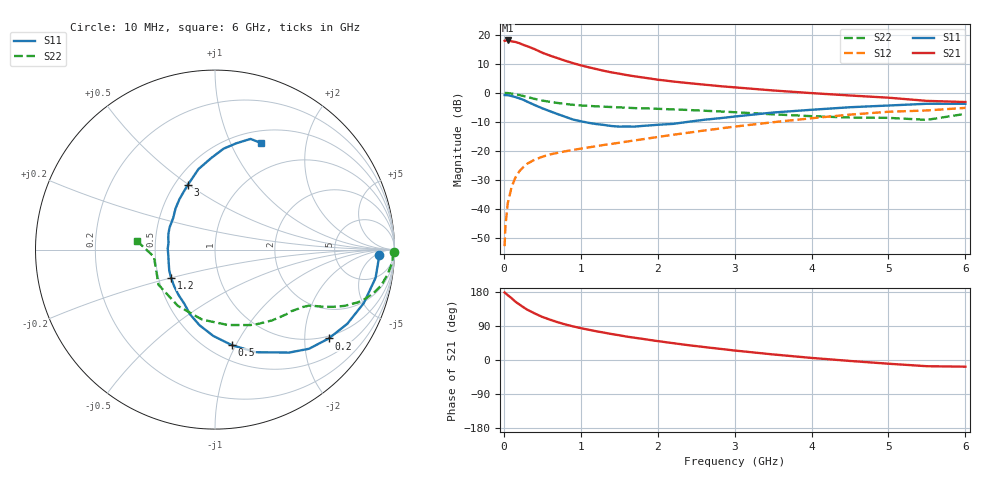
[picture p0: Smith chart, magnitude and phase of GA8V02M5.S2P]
! Infineon Technologies  Discrete & RF Semiconductors
! BF775
! Si NPN RF Bipolar Junction Transistor in SOT23
! VCE = 8 V  IC = 2.5 mA
! Common Emitter S-Parameters:  May  1996
# GHz  S  MA  R  50
!  f  S11  S21  S12  S22
! GHz  MAG  ANG  MAG  ANG  MAG  ANG  MAG  ANG
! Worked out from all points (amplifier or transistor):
!   36 points, 10 MHz to 6 GHz, reference 50 ohm
!   highest |S21| = 18.0 dB at 50 MHz (marker M1)
!   |S21| within 3 dB of that: start of sweep to 401 MHz
!   unconditionally stable (mu >= 1): 1.133 GHz to 3.189 GHz
!   at 250 MHz: K = 0.31, MSG = 21.1 dB, |S12| = -25.6 dB
!   at 1.4 GHz: K = 1.09, MAG = 10.5 dB, |S12| = -17.6 dB
!   at 6 GHz: K = 0.93, MSG = 1.0 dB, |S12| = -5.2 dB
!   S11 on the Smith chart (normalised r, x): 10 MHz: 20, -8; 200 MHz: 0.93, -2.61; 500 MHz: 0.64, -0.97; 1.2 GHz: 0.58, -0.20; 3 GHz: 0.58, +0.49; 6 GHz: 0.64, +1.31
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0.01  0.9151 -2.0  7.838 178.3  0.0023 91.4  0.9965 -0.8
0.02  0.9124 -4.1  7.905 176.2  0.005 86.0  0.9928 -1.7
0.05  0.9084 -10.0  7.952 171.3  0.0124 84.1  0.9894 -4.3
0.1  0.8809 -19.8  7.676 163.2  0.0238 79.9  0.9715 -8.2
0.15  0.845 -29.3  7.501 154.0  0.0348 73.2  0.9477 -12.1
0.2  0.8042 -38.0  7.151 146.8  0.0444 69.2  0.9157 -15.3
0.3  0.7073 -54.2  6.36 133.3  0.0598 62.2  0.8501 -20.2
0.4  0.6158 -68.2  5.638 123.0  0.0708 57.1  0.7865 -23.5
0.5  0.541 -79.9  4.889 113.7  0.0793 53.9  0.735 -25.7
0.6  0.4819 -91.0  4.365 106.4  0.0871 51.9  0.6995 -27.1
0.7  0.4299 -101.6  3.942 99.7  0.0927 50.6  0.6683 -28.3
0.8  0.3861 -111.2  3.554 93.8  0.0986 49.9  0.6429 -29.3
0.9  0.3465 -119.6  3.235 88.7  0.1042 50.2  0.6218 -30.1
1.1  0.3048 -138.6  2.755 80.0  0.115 50.6  0.596 -32.1
1.2  0.2903 -147.6  2.565 75.9  0.1204 50.7  0.5853 -33.1
1.6  0.2634 178.9  2.015 61.6  0.1449 52.3  0.5541 -37.7
2.2  0.292 142.9  1.565 44.4  0.1895 53.2  0.5182 -47.2
3  0.3905 112.9  1.241 25.0  0.262 49.9  0.4639 -65.0
3.5  0.4579 101.6  1.097 14.7  0.3118 45.8  0.4262 -80.3
4.5  0.5646 85.1  0.899 -2.5  0.4213 34.4  0.3756 -123.5
5.5  0.6477 72.2  0.726 -16.4  0.4972 18.1  0.3425 -173.3
6  0.6469 66.5  0.694 -17.6  0.5503 13.6  0.4344 173.9
